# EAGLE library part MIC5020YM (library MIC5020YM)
MICROCHIP - MIC5020YM - IC, DRIVER, MOSFET, LOW SIDE Source: Datasheet
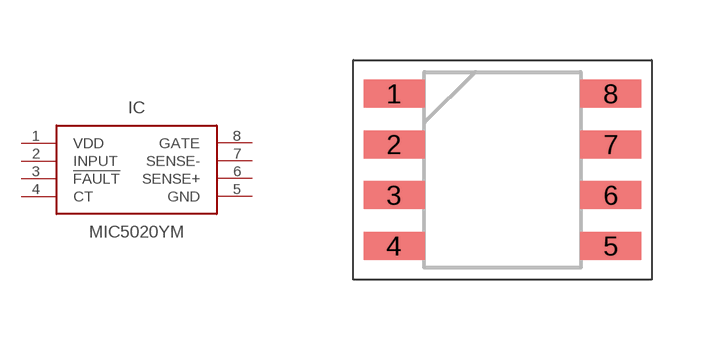
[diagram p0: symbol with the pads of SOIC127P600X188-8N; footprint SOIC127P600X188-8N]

Designator prefix IC

## MIC5020YM (Description: MICROCHIP - MIC5020YM - IC, DRIVER, MOSFET, LOW SIDE; Height: 1.879mm; Manufacturer_Name: Microchip; Manufacturer_Part_Number: MIC5020YM; RS_Part_Number: 9101537; Supplier_Name: RS)  [SOIC127P600X188-8N]
1  VDD  pwr
2  INPUT  in
3  !FAULT  out
4  CT  pas
5  GND  pwr
6  SENSE+  pas
7  SENSE-  pas
8  GATE  out

## Footprint SOIC127P600X188-8N (pad centres in mm)
8-Lead SOIC (M)
smd 1.525 x 0.7: 1 -2.712,1.905; 2 -2.712,0.635; 3 -2.712,-0.635; 4 -2.712,-1.905; 5 2.712,-1.905; 6 2.712,-0.635; 7 2.712,0.635; 8 2.712,1.905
